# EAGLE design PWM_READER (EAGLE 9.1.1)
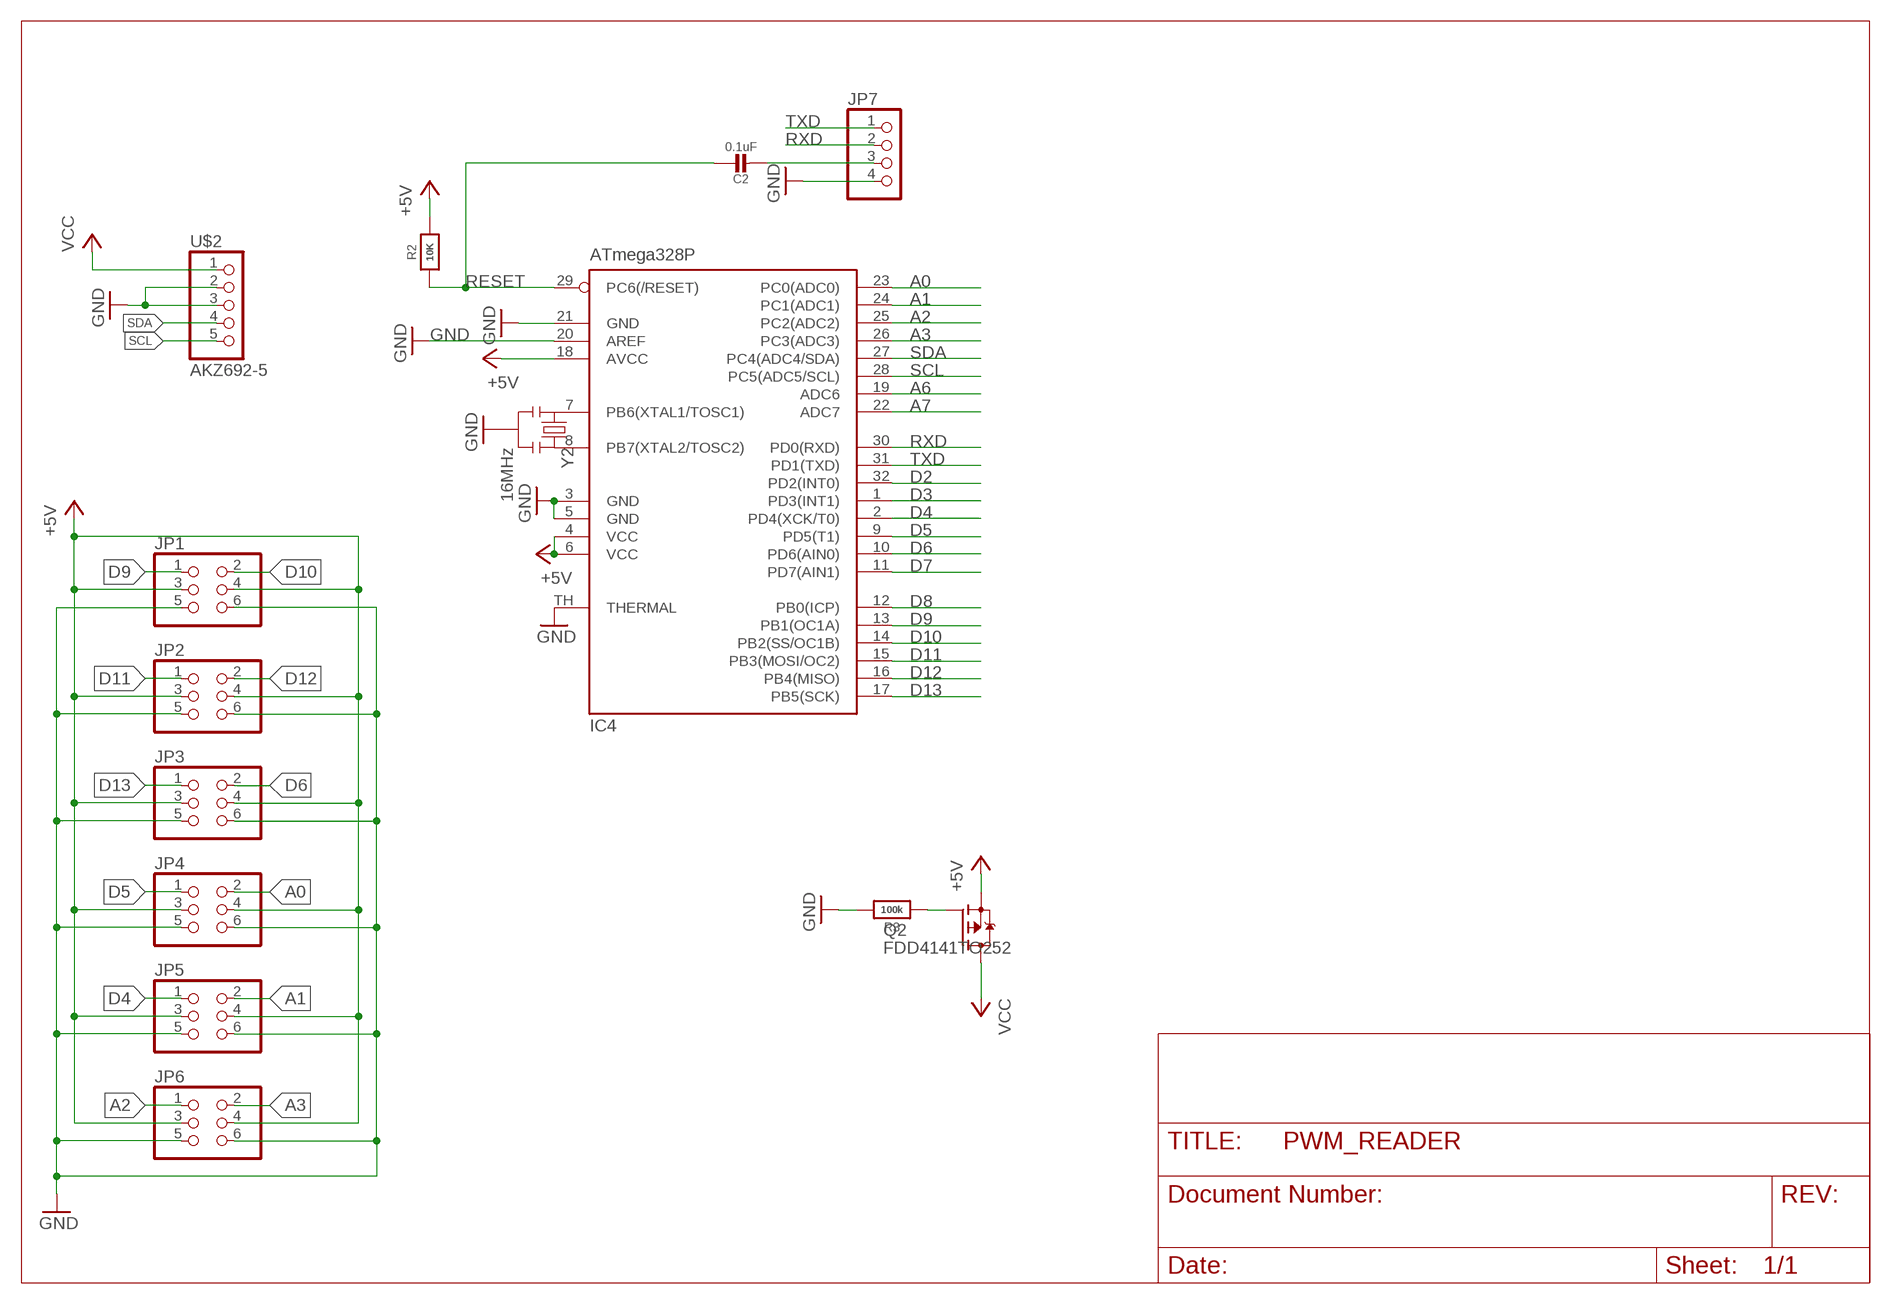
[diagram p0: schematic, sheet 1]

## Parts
C2  0.1uF  CAP_CERAMIC0805-NOOUTLINE  [0805-NO]
IC4  ATmega328P  MEGA8-MI  [MLF32-TH]
JP1  PINHD-2X3  [2X03]
JP2  PINHD-2X3  [2X03]
JP3  PINHD-2X3  [2X03]
JP4  PINHD-2X3  [2X03]
JP5  PINHD-2X3  [2X03]
JP6  PINHD-2X3  [2X03]
JP7  PINHD-1X4  [1X04]
Q2  FDD4141TO252  [TO252]
R2  10K  RESISTOR0805_NOOUTLINE  [0805-NO]
R3  100k  RESISTOR0805_NOOUTLINE  [0805-NO]
U$2  AKZ692-5  [1X5]
Y2  16MHz  RESONATORSMD  [RESONATOR-SMD]

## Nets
+5V: IC4.4(VCC) IC4.6(VCC) IC4.18(AVCC) JP1.3 JP1.4 JP2.3 JP2.4 JP3.3 JP3.4 JP4.3 JP4.4 JP5.3 JP5.4 JP6.3 JP6.4 Q2.2(S) R2.2
A0: IC4.23(PC0(ADC0)) JP4.2
A1: IC4.24(PC1(ADC1)) JP5.2
A2: IC4.25(PC2(ADC2)) JP6.1
A3: IC4.26(PC3(ADC3)) JP6.2
A6: IC4.19(ADC6)
A7: IC4.22(ADC7)
D2: IC4.32(PD2(INT0))
D3: IC4.1(PD3(INT1))
D4: IC4.2(PD4(XCK/T0)) JP5.1
D5: IC4.9(PD5(T1)) JP4.1
D6: IC4.10(PD6(AIN0)) JP3.2
D7: IC4.11(PD7(AIN1))
D8: IC4.12(PB0(ICP))
D9: IC4.13(PB1(OC1A)) JP1.1
D10: IC4.14(PB2(SS/OC1B)) JP1.2
D11: IC4.15(PB3(MOSI/OC2)) JP2.1
D12: IC4.16(PB4(MISO)) JP2.2
D13: IC4.17(PB5(SCK)) JP3.1
DTR/RTS1: C2.2 JP7.3
GND: IC4.3(GND) IC4.5(GND) IC4.20(AREF) IC4.21(GND) IC4.TH(THERMAL) JP1.5 JP1.6 JP2.5 JP2.6 JP3.5 JP3.6 JP4.5 JP4.6 JP5.5 JP5.6 JP6.5 JP6.6 JP7.4 R3.2 U$2.2 U$2.3 Y2.2
N$7: IC4.8(PB7(XTAL2/TOSC2)) Y2.3
N$8: IC4.7(PB6(XTAL1/TOSC1)) Y2.1
N$62: Q2.1(G) R3.1
RESET: C2.1 IC4.29(PC6(/RESET)) R2.1
RXD: IC4.30(PD0(RXD)) JP7.2
SCL: IC4.28(PC5(ADC5/SCL)) U$2.5
SDA: IC4.27(PC4(ADC4/SDA)) U$2.4
TXD: IC4.31(PD1(TXD)) JP7.1
VCC: Q2.3(D) U$2.1

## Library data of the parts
C2 = microbuilder:CAP_CERAMIC: Ceramic Capacitors
IC4 = microbuilder:MEGA8-MI: MICROCONTROLLER 8 Kbytes FLASH, 1 kbytes SRAM, 512 bytes EEPROM, USART, 6-channel 10 bit ADC, 2-channel 8 bit ADC Pin compatible with Atmega48, ATMega88, ATMega168 Source: avr.lbr; MPN: ATMEGA88PA-MU; OC_FARNELL: 1715491; OC_NEWARK: 15R0272
JP1-JP6 = pinhead:PINHD-2X3: PIN HEADER
JP7 = pinhead:PINHD-1X4: PIN HEADER
Q2 = transistor-fet:FDD4141: P-Channel PowerTrench® MOSFET Source: FDD4141.pdf
R2 R3 = microbuilder:RESISTOR: Resistors
U$2 = HeRo:AKZ692-5
Y2 = SparkFun:RESONATOR: Resonator Small SMD resonator. This is the itty bitty 10/20MHz resonators with built in caps. CSTCE10M0G55 and CSTCE20M0V53. Footprint has been reviewed closely but hasn't been tested yet.

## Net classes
1 power: width 0.305 mm

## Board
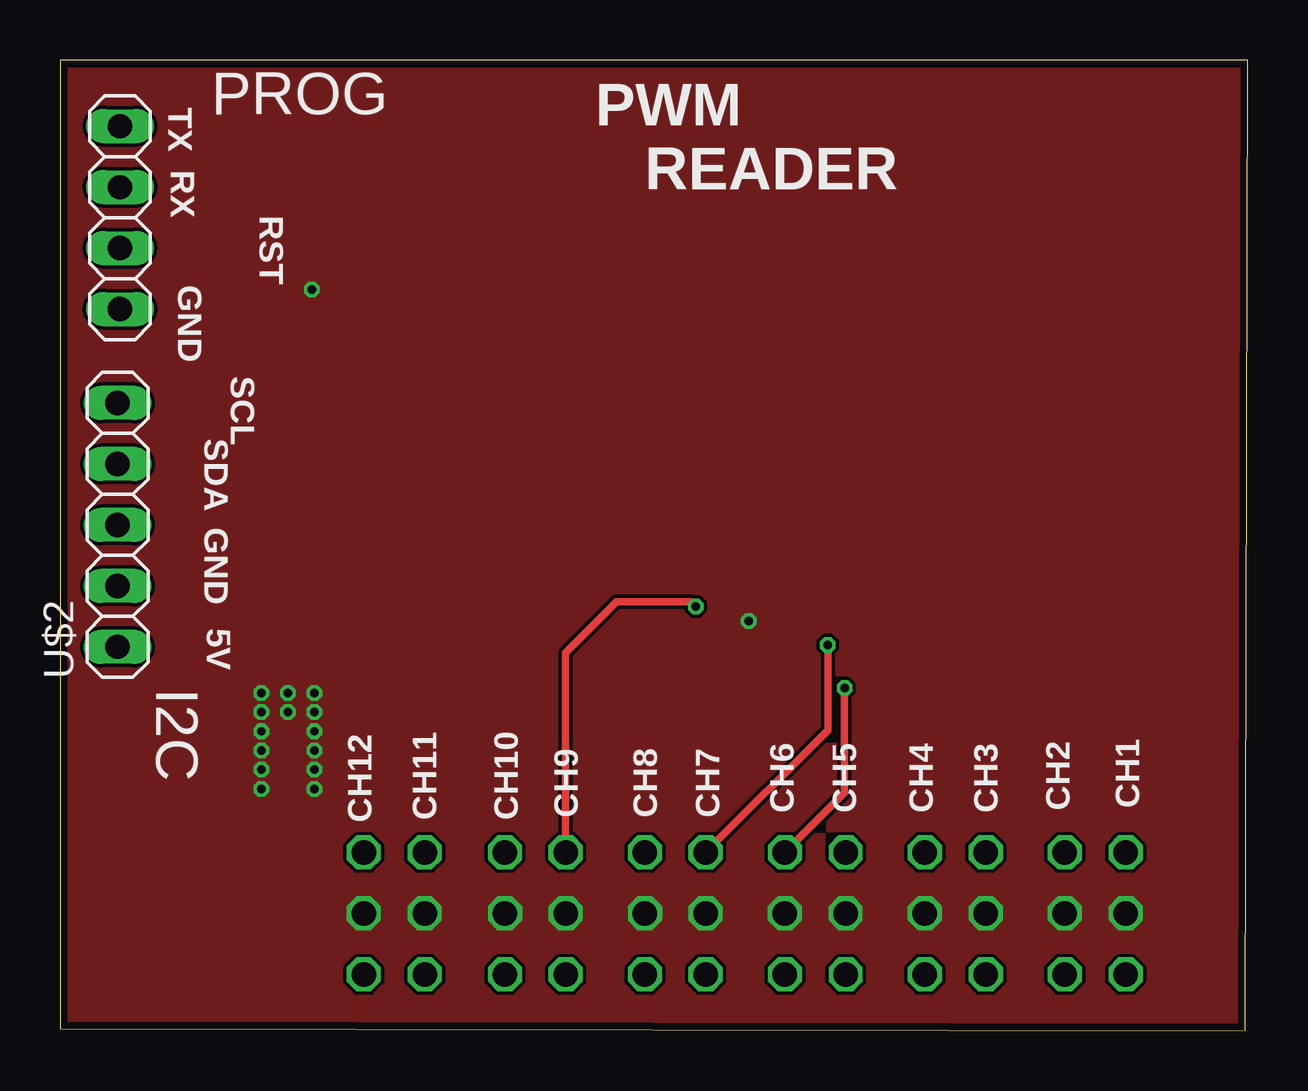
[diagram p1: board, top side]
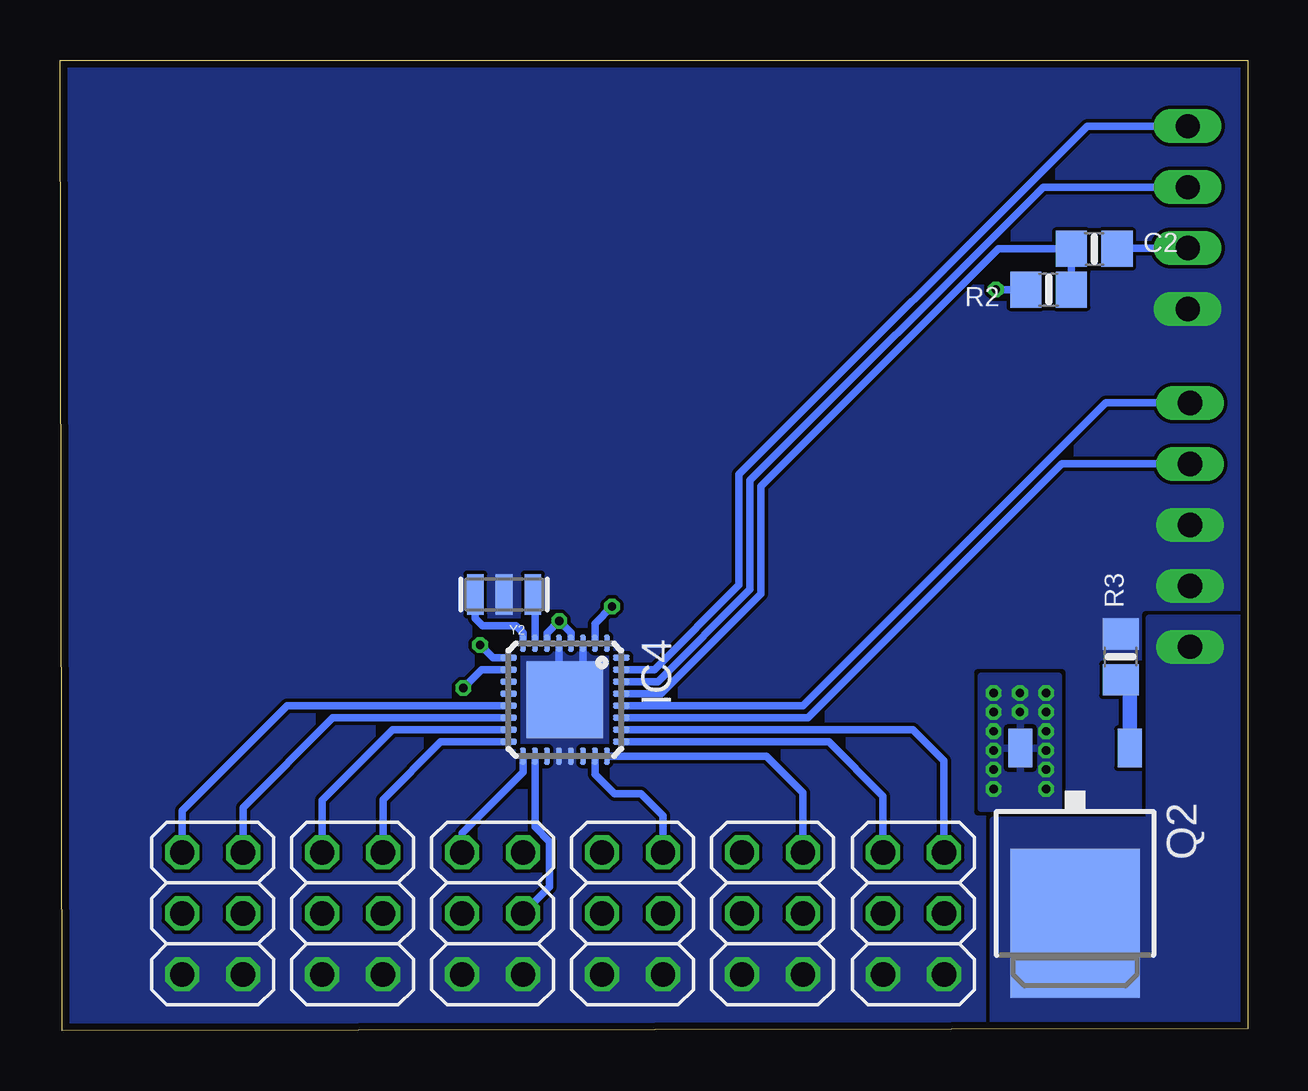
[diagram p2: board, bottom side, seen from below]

Size 49.51 x 40.44 mm. Coordinates in mm from the lower left corner, seen from the top.
Outline: 0,0.07 49.41,0 49.51,40.44 0,40.44 0,0.07
Copper layers (1*16): Top 0.035mm / dielectric 1.5mm / Bottom 0.035mm
Design rules "PCB-POOL Standard": minimum track width 0.15mm, minimum drill 0.3mm, track to track 0.15mm, track to pad 0.15mm, pad to pad 0.15mm, via to via 0.15mm, smd to smd 0.15mm, copper to edge 0.3mm, drill to drill 0.2mm, minimum pad ring 0.2mm, minimum via ring 0.15mm, stop-mask expansion 0.075mm, vias tented up to drill 0mil, thermal gap 0.2mm

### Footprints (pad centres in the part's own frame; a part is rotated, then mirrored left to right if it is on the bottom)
0805-NO = smd 1.3 x 1.5: 1 -0.95,0; 2 0.95,0
MLF32-TH = smd 0.7 x 0.25: 1 -2.35,1.75; 2 -2.35,1.25; 3 -2.35,0.75; 4 -2.35,0.25; 5 -2.35,-0.25; 6 -2.35,-0.75; 7 -2.35,-1.25; 8 -2.35,-1.75; 17 2.35,-1.75; 18 2.35,-1.25; 19 2.35,-0.75; 20 2.35,-0.25; 21 2.35,0.25; 22 2.35,0.75; 23 2.35,1.25; 24 2.35,1.75 | smd 0.25 x 0.7: 9 -1.75,-2.35; 10 -1.25,-2.35; 11 -0.75,-2.35; 12 -0.25,-2.35; 13 0.25,-2.35; 14 0.75,-2.35; 15 1.25,-2.35; 16 1.75,-2.35; 25 1.75,2.35; 26 1.25,2.35; 27 0.75,2.35; 28 0.25,2.35; 29 -0.25,2.35; 30 -0.75,2.35; 31 -1.25,2.35; 32 -1.75,2.35 | smd 3.2 x 3.2: TH 0,0
2X03 = drill 1.016 octagon: 1 -2.54,-1.27; 2 -2.54,1.27; 3 0,-1.27; 4 0,1.27; 5 2.54,-1.27; 6 2.54,1.27
1X04 = drill 1.016 long: 1 -3.81,0; 2 -1.27,0; 3 1.27,0; 4 3.81,0
TO252 = smd 1 x 1.6: 1 -2.28,-4.8; 2 2.28,-4.8 | smd 5.4 x 6.2: 3 0,2.5
1X5 = drill 1.016 long: 1 -5.08,0; 2 -2.54,0; 3 0,0; 4 2.54,0; 5 5.08,0
RESONATOR-SMD = smd 0.7 x 1.7: 1 -1.2,0; 2 0,0; 3 1.2,0

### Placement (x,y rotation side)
C2  6.4,32.57 0 bottom
IC4  28.47,13.78 270 bottom
JP1  43.15,4.88 270 bottom
JP2  37.31,4.88 270 bottom
JP3  31.48,4.88 270 bottom
JP4  25.65,4.88 270 bottom
JP5  19.81,4.88 270 bottom
JP6  13.93,4.88 270 bottom
JP7  2.5,33.87 270 top
Q2  7.2,6.97 180 bottom
R2  8.3,30.87 180 bottom
R3  5.3,15.57 90 bottom
U$2  2.4,21.07 90 top
Y2  31,18.17 180 bottom

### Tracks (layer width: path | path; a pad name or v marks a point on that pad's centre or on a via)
+5V  (via drill 0.35)
  Bottom 0.305: IC4.6 29.22,16.55 v28.7,17.07 28.22,16.59 IC4.4 | IC4.18 29.72,8.49 29.1,7.87 29.1,5.99 JP3.4 | v10.5,30.87 R2.2
  other vias: 8.4,12.47 8.4,11.67 8.4,10.87 8.4,10.07 8.4,13.27 8.4,14.07 9.5,14.07 10.6,14.07 9.5,13.27 10.6,13.27 10.6,12.47 10.6,11.67 10.6,10.87 10.6,10.07
  pour Top (no thermals): 0,40.44 49.53,40.44 49.53,0.07 0,0.07
  pour Bottom: 7.9,14.77 11.1,14.77 11.1,9.27 7.9,9.27
A0
  Bottom 0.305: IC4.23 27.22,10.69 26.4,9.87 25.3,9.87 24.38,8.95 JP4.2
A1
  Bottom 0.305: IC4.24 20.06,11.43 18.54,9.91 JP5.2
A2
  Bottom 0.305: IC4.25 17.46,12.03 15.2,9.77 JP6.1
A3
  Bottom 0.305: IC4.26 13.96,12.53 12.66,11.23 JP6.2
D4  (via drill 0.35)
  Top 0.305: JP5.1 21.08,15.75 23.2,17.87 26.3,17.87 v26.5,17.67
  Bottom 0.305: v26.5,17.67 27.22,16.95 IC4.2
D5  (via drill 0.35)
  Top 0.305: JP4.1 32,12.5 v32,16.07
  Bottom 0.305: v32,16.07 31.46,15.53 IC4.9
D6  (via drill 0.35)
  Top 0.305: JP3.2 32.7,9.91 v32.7,14.27
  Bottom 0.305: v32.7,14.27 31.94,15.03 IC4.10
D9
  Bottom 0.305: IC4.13 40.04,13.53 44.42,9.15 JP1.1
D10
  Bottom 0.305: IC4.14 38.14,13.03 41.88,9.29 JP1.2
D11
  Bottom 0.305: IC4.15 35.64,12.53 38.58,9.59 JP2.1
D12
  Bottom 0.305: IC4.16 33.64,12.03 36.04,9.63 JP2.2
D13
  Bottom 0.305: IC4.17 30.22,10.75 32.75,8.22 JP3.1
DTR/RTS1
  Bottom 0.305: C2.2 5.42,32.6 JP7.3
GND
  Bottom 0.305: IC4.5 28.72,14.03 IC4.TH 27.72,14.53 IC4.3
  pour Bottom (rank 2, no thermals): 0,40.44 49.53,40.44 49.53,0.07 0,0.07
N$7
  Bottom 0.305: IC4.8 30.22,16.59 30.5,16.87 31.9,16.87 32.2,17.17 Y2.3
N$8
  Bottom 0.305: IC4.7 29.72,18.09 Y2.1
N$62
  Bottom 0.61: Q2.1 4.92,14.24 R3.1
RESET
  Bottom 0.305: IC4.29 24.45,14.03 20.29,18.19 20.29,22.68 10.4,32.57 C2.1 R2.1
RXD
  Bottom 0.305: JP7.2 8.53,35.14 20.75,22.93 20.75,18.38 24.59,14.53 IC4.30
SCL
  Bottom 0.305: IC4.28 18.54,13.53 5.92,26.15 U$2.5
SDA
  Bottom 0.305: IC4.27 18.34,13.03 7.76,23.61 U$2.4
TXD
  Bottom 0.305: JP7.1 6.69,37.68 21.2,23.17 21.2,18.57 24.74,15.03 IC4.31
VCC
  pour Bottom (no thermals): 0,17.17 4.1,17.17 4.1,8.77 10.6,8.77 10.6,0.07 0,0.07

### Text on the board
tPlace: TX | PROG | RX | PWM / READER | RST | GND | SCL | SDA | GND | 5V | I2C | CH12 | CH11 | CH10 | CH9 | CH8 | CH7 | CH6 | CH5 | CH4 | CH3 | CH2 | CH1

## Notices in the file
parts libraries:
microbuilder: This work is placed in the public domain, and may be freely used for commercial and non-commercial work with the following conditions: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
SparkFun: Licensing: CC v3.0 Share-Alike You are welcome to use this library for commercial purposes.
